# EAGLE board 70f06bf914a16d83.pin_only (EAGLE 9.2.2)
REV: B

Size 22.86 x 22.86 mm. Coordinates in mm from the lower left corner, seen from the top.
Outline: 0,20.14 0,2.79 arc90 2.54,0 20.22,0 arc90 22.86,2.56 22.86,19.89 arc90 20.24,22.86 2.49,22.86 arc90 0,20.14
Copper layers (1*16): Top 0.035mm / dielectric 1.5mm / Bottom 0.035mm
Design rules "adafruit": minimum track width 8mil, minimum drill 15.5mil, track to track 8mil, track to pad 8mil, pad to pad 8mil, via to via 8mil, smd to smd 8mil, copper to edge 10mil, drill to drill 8mil, minimum pad ring 10mil, minimum via ring 8mil, stop-mask expansion 2mil, vias tented up to drill 20mil, thermal gap 10mil

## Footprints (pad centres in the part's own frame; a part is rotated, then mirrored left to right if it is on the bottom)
0603-NO = smd 1.075 x 1: 1 -0.85,0; 2 0.85,0
MICROBUILDER_FIDUCIAL_1MM = smd 1 x 1: 1 0,0
TSSOP16 = smd 0.305 x 0.991: 1 -2.275,-2.918; 2 -1.625,-2.918; 3 -0.975,-2.918; 4 -0.325,-2.918; 5 0.325,-2.918; 6 0.975,-2.918; 7 1.625,-2.918; 8 2.275,-2.918; 9 2.275,2.918; 10 1.625,2.918; 11 0.975,2.918; 12 0.325,2.918; 13 -0.325,2.918; 14 -0.975,2.918; 15 -1.625,2.918; 16 -2.275,2.918
1X08_ROUND_70 = drill 1 pad 1.778: 1 -8.89,0; 2 -6.35,0; 3 -3.81,0; 4 -1.27,0; 5 1.27,0; 6 3.81,0; 7 6.35,0; 8 8.89,0
SOLDERJUMPER_CLOSEDWIRE = smd 1.168 x 1.6: 1 -0.762,0; 2 0.762,0 | smd 0.635 x 0.203: WIRE 0,0
SOLDERJUMPER_ARROW_NOPASTE = smd 0.762 x 1.524: 1 -1.016,0; 2 1.016,0
TESTPOINT_ROUND_1.5MM = smd 1.5 x 1.5: P$1 0,0
MOUNTINGHOLE_2.5_PLATED = drill 2.5 pad 3.2: P$1 0,0
TERMBLOCK_508_1X2 = drill 1.1 pad 2.184 long: P$3 -2.54,0; P$4 2.54,0

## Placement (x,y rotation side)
C1  1uF  [0603-NO]  15.76,6.65 270 top
FID3  MICROBUILDER_FIDUCIAL""  [MICROBUILDER_FIDUCIAL_1MM]  20.32,5.49 0 top
FID4  MICROBUILDER_FIDUCIAL""  [MICROBUILDER_FIDUCIAL_1MM]  1.22,17.45 0 top
IC1  INA260  [TSSOP16]  11.43,10.16 270 top
JP2  [1X08_ROUND_70]  11.43,2.54 0 top
R1  10K  [0603-NO]  8.23,6.15 180 top
R2  10K  [0603-NO]  13.45,6.53 0 top
R3  10K  [0603-NO]  3.5,7.42 180 top
R4  10K  [0603-NO]  3.5,8.94 180 top
SJ1  [SOLDERJUMPER_CLOSEDWIRE]  17.53,8.38 90 top
SJ3  [SOLDERJUMPER_ARROW_NOPASTE]  3.56,5.79 0 top
SJ4  [SOLDERJUMPER_ARROW_NOPASTE]  3.56,10.62 0 top
TP1  [TESTPOINT_ROUND_1.5MM]  3.56,9.78 0 bottom
TP2  [TESTPOINT_ROUND_1.5MM]  3.56,5.84 0 bottom
U$1  [ADAFRUIT_3.5MM]  18.8,10.41 90 top
U$6  [PCBFEAT-REV-040]  11.43,21.34 0 bottom
U$7  MOUNTINGHOLE2.5  [MOUNTINGHOLE_2.5_PLATED]  20.32,20.32 0 top
U$8  MOUNTINGHOLE2.5  [MOUNTINGHOLE_2.5_PLATED]  2.54,20.32 0 top
X1  5.08mm Term  [TERMBLOCK_508_1X2]  11.43,19.05 0 top

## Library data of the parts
C1 IC1 JP2 R1-R4 SJ1 TP1 TP2 U$1 U$6 X1 = microbuilder
FID3 FID4 = Adafruit_INA219_CurPowerMonitor
SJ3 SJ4 U$7 U$8 = microbuilder; BOM: EXCLUDE

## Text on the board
tPlace: Vin+ | Vin- | I2C / Addr | A1 | INA260 / Power Sensor | VB | A0 | Vcc | SCL | Alert | Vin+ | GND | SDA | VBus | Vin-
bPlace: INA260 Precision DC / Current/Power Monitor | Bus Voltage: 0-36V | Max Current: 15A | VCC/Logic: 3-5V

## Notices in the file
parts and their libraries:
microbuilder: This work is placed in the public domain, and may be freely used for commercial and non-commercial work with the following conditions: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
